(* Logix 5000 Rung export; software revision 16.04 *)

TYPE AFCESiteAlarms :   // Indicates if a meter has any alarms
STRUCT
   Meter1 : BOOL;   // Meter in alarm
   Meter2 : BOOL;   // Meter in alarm
   Meter3 : BOOL;   // Meter in alarm
   Meter4 : BOOL;   // Meter in alarm
   Meter5 : BOOL;   // Meter in alarm
   Meter6 : BOOL;   // Meter in alarm
   Meter7 : BOOL;   // Meter in alarm
   Meter8 : BOOL;   // Meter in alarm
   Meter9 : BOOL;   // Meter in alarm
   Meter10 : BOOL;   // Meter in alarm
   Meter11 : BOOL;   // Meter in alarm
   Meter12 : BOOL;   // Meter in alarm
   Meter13 : BOOL;   // Meter in alarm
   Meter14 : BOOL;   // Meter in alarm
   Meter15 : BOOL;   // Meter in alarm
   Meter16 : BOOL;   // Meter in alarm
END_STRUCT
END_TYPE

TYPE AFCEFlag :   // Flags contains status information updated by ladder and also trigger bits for clock update
STRUCT
   AFCStopped : BOOL;   // Indicates that the module has sent a new input block to be processed by ladder - UPDATED BY LADDER
   AFCInputSequenceNum : INT;   // Meter number (0 -15) associated to blocks 1-16. Used to update "Profile" (meter type and product group.) UPDATED BY LADDER
END_STRUCT
END_TYPE

TYPE AFCEUtilBlockNonInterrupt :
STRUCT
   Now : BOOL;
   ModbusMasterCommand : BOOL;
   ModbusMasterResponse : BOOL;
   Archive : DINT;
   Prover : BOOL;
   PassThru : BOOL;
   Calibration : BOOL;
END_STRUCT
END_TYPE

TYPE AFCEProveConfigEnable :   // Prove controls at enable
STRUCT
   MeterNumber : INT;   // Meter number requested (1-16)
   AutoAcceptProve : BOOL;   // Auto-accept the prove
   AutoContinueProve : BOOL;   // Auto-continue the prove
END_STRUCT
END_TYPE

TYPE AFCEModbusGateway :   // Modbus Gateway
STRUCT
   Command : AFCEModbusGatewayCommand[10];   // Modbus gateway commands - contains setup and modbus data
END_STRUCT
END_TYPE

TYPE AFCENetworkConfig :
STRUCT
   GatewayIndex : DINT;
   Physical_Interface_IP : INT[4];
   Physical_Interface_Network_Prefix : SINT;
   Default_Gateway_IP : INT[4];   // The IP address of the gateway. Must be in the same network as the web interface, or null.
   Server1_Network_Prefix : SINT;   // The network prefix length (number of subnet mask bits) of the interface for server 1; a number between 0 and 32.
   Server1_MBAP_Port : DINT;   // The Modbus-TCP port for server 1; 502, or a number between 1024 and 65535.
   Server1_Listener_IP : INT[4];   // The IP address of the network interface for server 1.
END_STRUCT
END_TYPE

TYPE AFCEModbusMasterDataType :   // Modbus master data type
STRUCT
   Bit : BOOL;   // bit type
   Word : BOOL;   // word type (16-bit)
   Long : BOOL;   // long integer (32-bit)
   LongRemote : BOOL;   // long integer (32-bit)
END_STRUCT
END_TYPE

TYPE AFCEUtil :   // Used for internal ladder logic usage. These values must not be changed by user application.
STRUCT
   Flags : AFCEFlag;   // Wallclock update commands
   CycleCounter : INT;   // Reflects current block ID calculated by ladder to be sent to the module
   Buffer : AFCEUtilBuffer;
   Block : AFCEUtilBlock;
END_STRUCT
END_TYPE

TYPE AFCEWallclock :
STRUCT
   GetAFCTime : BOOL;   // Get current AFC Time
   SetAFCTimeFromPLCTime : BOOL;   // Set AFC time from PLC time. Updates current AFC time
   EnableLocalDateTime : BOOL;   // Enable Local Date Time.
   AFCTime : AFCETime;   // Coordinated Universal Time. Updated by either getting or setting AFC time.
END_STRUCT
END_TYPE

TYPE AFCEProvePhaseBitmap :   // AFC prove phase bitmap
STRUCT
   NotSelected : BOOL;   // Not selected
   Active : BOOL;   // Active, not counting
   CountingPast1stSwitch : BOOL;   // Counting past 1st switch for Udir and forward leg for Bdir)
   Past2ndSwitchFwdLeg : BOOL;   // Past 2nd switch forward leg (bidirectional only)
   Past1stSwithRetLeg : BOOL;   // Past 1st switch return leg (bidirectional only)
   RunComplete : BOOL;   // Run complete. past 2nd switch.
END_STRUCT
END_TYPE

TYPE AFCEProveInputConfig :   // Prove input block results - prover configuration
STRUCT
   Type : INT;   // Prover type
   Options : INT;   // Prover options
   RunsPerProveTotal : INT;   // Total runs per prove
   RunsPerProveSelected : INT;   // Selected runs per prove
   MaxRunsBeforeAbort : INT;   // Max total runs before abort
   ShortPassesPerRun : INT;   // Short passes per run if bidir = 2 , else 0
END_STRUCT
END_TYPE

TYPE AFCEModbusGatewayCommand :   // Modbus Gateway Command
STRUCT
   Config : AFCEModbusGatewayConfig;   // Config data to be entered by the user.
   Trigger : BOOL;   // Trigger the Command, when cleared module has responded.
   Data : INT[200];   // Contains modbus data written to the module (write commands)
END_STRUCT
END_TYPE

TYPE AFCENetworkUTIL :
STRUCT
   State : INT;
   Buffer : SINT[240];
   TimeoutTimer : TIMER;
   TimeoutState : INT;
END_STRUCT
END_TYPE

TYPE AFCEProveConfigAccept :   // Prove controls at accept. If auto-accept is selected must be available at enable
STRUCT
   RequestedInterpolationPoint : INT;   // Requested interpolation point (0 nearest)
   ApplyMFChangeAllStreams : BOOL;   // Apply change in meter factor to all streams
   ApplyMFChangeCurve : BOOL;   // Apply change in meter factor to all curve points
   ApplyNewMF : BOOL;   // CApply new meter factor
END_STRUCT
END_TYPE

TYPE AFCEModbusMasterCommand :   // Modbus Master Command
STRUCT
   Config : AFCEModbusMasterConfig;   // Modbus Master Configuration
   ErrorCode : INT;   // Error Code associated to Modbus Master Command
   Pending : BOOL;   // Pending Modbus Master Command - waiting for Modbus Response
   ReturnedTransactionID : DINT;   // Changes to Config.TransactionID value when response has returned.
   Data : INT[100];   // Read or Write Data
END_STRUCT
END_TYPE

TYPE AFCEProveSequencing :   // AFC prove sequencing tag for phase selection and ball positioning
STRUCT
   Phase : AFCEProvePhaseBitmap;   // AFC phase sequencing
   BallPositionReady : BOOL;   // Ball position: Ready (Udir & Bdir only; fwd leg Bdir)
   BallPositionSealed : BOOL;   // Ball position: Sealed (Udir & Bdir only; fwd leg Bdir)
   BallPositionReadyBwdLeg : BOOL;   // Ball position: Ready bwd leg (Bdir only)
   BallPositionSealedBwdLeg : BOOL;   // Ball position: Sealed bwd leg (Bdir only)
END_STRUCT
END_TYPE

TYPE AFCEUtilBlockInterrupt :
STRUCT
   Now : BOOL;
   ModbusGateway : DINT;
   EnableDisable : BOOL;
   Analysis : DINT;
END_STRUCT
END_TYPE

TYPE AFCEUtilBlock :
STRUCT
   ProcessInput : INT;
   InterruptPending : AFCEUtilBlockInterrupt;
   InterruptComplete : AFCEUtilBlockInterrupt;
   NonInterruptPending : AFCEUtilBlockNonInterrupt;
   NonInterruptComplete : AFCEUtilBlockNonInterrupt;
END_STRUCT
END_TYPE

TYPE AFCEModbusGatewayConfig :   // Modbus Ggateway Configuration
STRUCT
   Enable : BOOL;   // Set to 1 to enable modbus gateway command (0=disable)
   StartRegister : DINT;   // Start modbus address
   RegisterCount : INT;   // Word count (200 max)
   FunctionType : BOOL;   // 0 = read command, 1 = write command
   RegisterType : BOOL;   // 0 = holding register, 1 = input register
   SlaveType : BOOL;   // 0 = primary slave, 1 = virtual slave
END_STRUCT
END_TYPE

TYPE AFCENetwork :
STRUCT
   Read : BOOL;   // Trigger to read network parameters
   Write : BOOL;   // Trigger to write network parameters
   Config : AFCENetworkConfig;   // Network parameters
   Error : INT;   // 0 = OK, -1 = Timeout, -2 = Gateway Index Out of Range
   Util : AFCENetworkUTIL;   // Internal variables
END_STRUCT
END_TYPE

TYPE AFCEModbusPassThru :   // AFC Modbus Pass-thru
STRUCT
   Enable : BOOL;   // Set to 1 to enable pass-thru functionality (requires AFC Manager setting)
   MessagePresent : BOOL;   // Message present in the response block
   GetMessage : BOOL;   // Get the pass-thru message. When the bit is cleared the message has been transferred to the PLC.
   FunctionBitWrite : BOOL;   // Function bit write
   OverflowError : BOOL;   // Overflow error flag
   ModbusAddress : INT;   // Destination modbus address
   RegisterCount : INT;   // Number of elements associated to command
   ReadDataWord : INT[125];   // Contains received data for word commands
   ReadDataBit : AFCEModbusPassThruBitData;   // Contains received data for bit commands
END_STRUCT
END_TYPE

TYPE AFCEUtilBuffer :   // Buffer
STRUCT
   Input : INT[248];   // Input buffer contains the complete block to be copied from the module
   Output : INT[247];   // Output buffer contains data the complete block to be copied to the module
   Process : INT[180];
   ArchiveDay : INT[98];
   ArchiveHour : INT[98];
   Prove : INT[26];
   Analysis : INT[198];
   MeterEnableDisable : INT[4];
   StreamEnable : INT[36];
   StreamDisable : INT[36];
   StreamSelect : INT[24];
   MeterSignals : INT[24];
   Calibration : INT[36];
END_STRUCT
END_TYPE

TYPE AFCEProveStatus :   // Status of the prove (returned from the module to the processor)
STRUCT
   ProveAccepted : BOOL;   // Prove was accepted
   MeterFactorApplied : BOOL;   // Meter factor was applied
   MFAppliedToCurve : BOOL;   // Meter factor was applied to all points in the curve
   MFAppliedToStreams : BOOL;   // Meter factor was applied to all streams
   ProveRejectedByCommand : BOOL;   // Prove was rejected by command
   ProveRejectedNoRuns : BOOL;   // Prove was rejected - empty prove (no runs)
   ProveRejectedDivideBy0 : BOOL;   // Prove was rejected - divide by 0
   ProveEnabled : BOOL;   // Prove is enabled
   ProvingRunInProgress : BOOL;   // Proving run is in progress
   ProveRejectedAbort : BOOL;   // Prove rejected: abort
   ProvePaused : BOOL;   // Prove is paused
   RunCancelled : BOOL;   // Run Is cancelled
   RunTimedOut : BOOL;   // Run timed out
END_STRUCT
END_TYPE

TYPE AFCEProveConfig :   // Controls (configuration settings) associated to the prover
STRUCT
   Enable : AFCEProveConfigEnable;   // Controls at enable
   Accept : AFCEProveConfigAccept;   // Controls at accept
END_STRUCT
END_TYPE

TYPE AFCESiteStatus :   // Site status bits - contains general information about the module - not meter specific
STRUCT
   AFCActive : BOOL;   // AFC active
   ChecksumAlarms : BOOL;   // Checkum alarm active
   Reserved2 : BOOL;
   Reserved3 : BOOL;
   PLCHalted : BOOL;   // PLC in program mode or missing
   CfgChanged : BOOL;   // Configuration changed
   Powerup : BOOL;   // Module powered up
   ColdStart : BOOL;   // Module performed cold start (BBRAM initialized)
   ModbusMasterPending : BOOL;   // Modbus Master Poll Pending
   ModbusMasterComplete : BOOL;   // Modbus Master Poll Complete
   ModbusPassThruPending : BOOL;   // Modbus Pass-thru Input Pending
   CalibrationRequest : BOOL;   // Calibration request from module
   ProverEnabled : BOOL;   // Prover Enabled
   Reserved13 : BOOL;
   Reserved14 : BOOL;
   Reserved15 : BOOL;
END_STRUCT
END_TYPE

TYPE AFCEModbusMaster :   // Modbus Master. Port 3 must be configured as modbus master through AFC Manager to use this feature.
STRUCT
   Enable : BOOL;   // Enable the modbus master funcionality
   CommandIndex : INT;   // Selects which command index will be executed
   Command : AFCEModbusMasterCommand[10];   // Each command contains a specific modbus request to be sent out of the port
END_STRUCT
END_TYPE

TYPE AFCEProveProcess :   // Prove process output from processor to the module
STRUCT
   Sequencing : AFCEProveSequencing;   // Prover sequencing
   Temperature : REAL;   // Temperature for Single Probe provers. And Inlet Temperature for Dual Probe Provers.
   OutletTemperature : REAL;   // Outlet Temperature for Provers with Dual Probes.
   SwitchBarTemperature : REAL;   // Switch bar temperature
   Pressure : REAL;   // Pressure for Single Probe provers. And Inlet Pressure for Dual Probe Provers.
   OutletPressure : REAL;   // Outlet Pressure for Provers with Dual Probes.
   ProverDensity : REAL;   // Prover density
END_STRUCT
END_TYPE

TYPE AFCETime :   // AFC time format used for wallclock update.
STRUCT
   Year : DINT;   // Year
   Month : DINT;   // Month
   Day : DINT;   // Day
   Hour : DINT;   // Hour
   Minute : DINT;   // Minute
   second : DINT;   // Seconds
END_STRUCT
END_TYPE

TYPE AFCEModbusMasterSwap :   // Modbus master swap words/ swap bytes
STRUCT
   SwapWords : BOOL;   // Swap words
   SwapBytes : BOOL;   // Swap bytes
END_STRUCT
END_TYPE

TYPE AFCEProvePulseCount :   // Values to be supplied at the end of the pass/run
STRUCT
   Meter : DINT;   // Meter pulse count
   MasterMeter : DINT;   // Master meter pulse count
END_STRUCT
END_TYPE

TYPE AFCEModbusPassThruBitData :   // AFC Modbus Pass-thru Bit Data
STRUCT
   Data : BOOL[2016];   // Contains received data for bit commands
END_STRUCT
END_TYPE

TYPE AFCEModbusMasterConfig :   // Modbus master command settings
STRUCT
   Enable : BOOL;   // Set to 1 to enable command (0=disable)
   FunctionType : BOOL;   // Set to 1 to select write command (0=read command)
   RegisterBank : BOOL;   // Set to 1 to select input register (0=holding register)
   DataType : AFCEModbusMasterDataType;   // Select data type format
   SwapOption : AFCEModbusMasterSwap;   // Select byte and word swap (1 = swap, 0 = no swap)
   TypeSwap : INT;   // This value is calculated by ladder logic and must not be modified by user
   SlaveAddress : INT;   // Modbus slave address of remote device
   ModbusAddress : INT;   // Modbus data address on remote slave
   ElementCount : INT;   // Number of data elements (125 words)
   TransactionID : INT;   // Transaction ID. This value is returned to the ReturnedTransaction ID when the response has been received.
END_STRUCT
END_TYPE

TYPE AFCEModuleDef :   // Main user defined data type
STRUCT
   ModbusGateway : AFCEModbusGateway;   // Reads and write data between processor and module modbus table
   ModbusMaster : AFCEModbusMaster;   // Setup modbus master commands to be sent to remote slaves (through Port 3)
   ModbusPassThru : AFCEModbusPassThru;   // Modbus pass-thru data
   SiteStatus : AFCESiteStatus;   // Site status
   MeterAlarms : AFCESiteAlarms;   // Meter Alarms
   Prove : AFCEProve;   // Prover
   Wallclock : AFCEWallclock;   // Set clock and get clock information
   Firmware : AFCEFirmwareVersion;   // Firmware information
   Util : AFCEUtil;   // Used by ladder logic
END_STRUCT
END_TYPE

TYPE AFCEProveSignals :   // Contains the proving signals that will trigger specific tasks from the module
STRUCT
   EnableProve : BOOL;   // Enables the prove
   AcceptProve : BOOL;   // Accepts the prove
   RejectProve : BOOL;   // Reject the prove
   RunStart : BOOL;   // Starts the run
   RunComplete : BOOL;   // Flags that the run is complete
   RunCancel : BOOL;   // Cancels the run
   RunDelete : BOOL;   // Deletes the run
   PassComplete : BOOL;   // Flag that the pass is complete
   PauseProve : BOOL;   // Pauses the Proving Process
   AbortProve : BOOL;   // Aborts the prove
END_STRUCT
END_TYPE

TYPE AFCEFirmwareVersion :
STRUCT
   Major : SINT;   // Major Version number
   Minor : SINT;   // Minor Version number
   Revision : INT;   // Revision
END_STRUCT
END_TYPE

TYPE AFCEProveRunResults :   // Run results of the prove. Copied from the module to the pocessor
STRUCT
   CountAttempted : INT;   // Run count attempted
   CountCompleted : INT;   // Run count completed
   CountSelected : INT;   // Run count selected
   RunsSelected : INT;   // Bit Mapped Runs selected for calculations from completed runs
   NewMeterFactor : REAL;   // New meter factor
   ChangeInMeterFactor : REAL;   // Change in meter factor
END_STRUCT
END_TYPE

TYPE AFCEProve :   // Prove
STRUCT
   Process : AFCEProveProcess;   // Process Variables
   Signals : AFCEProveSignals;   // AFC Prove Signals (triggers the proving update)
   Config : AFCEProveConfig;   // AFC Prove Control (configuration settings)
   PulseCounts : AFCEProvePulseCount;   // Pulse counts to be updated at the end of the run/pass
   ConfigInput : AFCEProveInputConfig;   // AFC prover input configuration
   Status : AFCEProveStatus;   // AFC prover status
   ErrorCode : INT;   // Prove error code
   ProveControlsEcho : INT;   // AFC module Echos the state of the Prove Controls
   RequestedMeterEcho : INT;   // AFC module Echos the Meter number requested
   RequestedCurvePointEcho : INT;   // AFC module Echos the requested Curve Point
   RunResults : AFCEProveRunResults;   // Prove and run results
   ProveEnabled : BOOL;   // ON if prove is enabled. This flag is coped from inputbuffer[247]
END_STRUCT
END_TYPE

ADD_ON_INSTRUCTION AOI69EAFCNetworkConfig   (* revision 1.0, ExecutePrescan *)
// Add-On instruction to update the MVI69E-AFC network settings
// Revision note:
// Read and write module network configuration.
// Help:
// v1.0 Read and write module network configuration.
VAR_IN_OUT
   Network : AFCENetwork; {required}
   EAFC : AFCEModuleDef; {required}
END_VAR
VAR
   NetworkBuffer : DINT[2];
   MVMbuffer : INT;
   IndexSizeM1 : DINT;
   IndexSize : DINT;
   Index : DINT;
   ErrorTimer : TIMER;
END_VAR

ROUTINE Logic   (* ladder *)
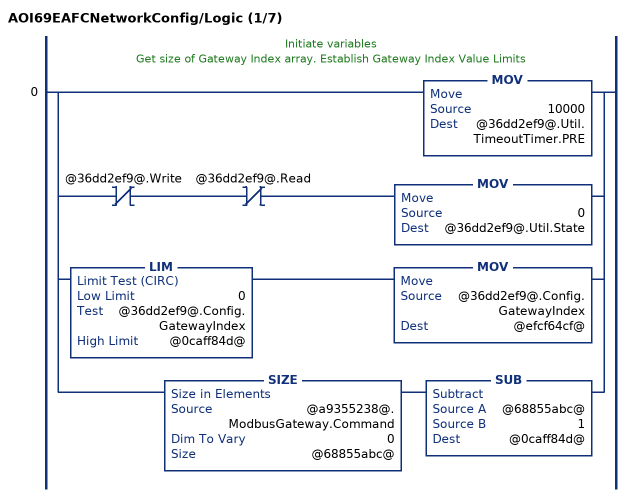
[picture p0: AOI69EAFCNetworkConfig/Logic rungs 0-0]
   // Initiate variables
   // Get size of Gateway Index array. Establish Gateway Index Value Limits
   0: [[MOV(10000,@36dd2ef9@.Util.TimeoutTimer.PRE) ,XIO(@36dd2ef9@.Write) XIO(@36dd2ef9@.Read) MOV(0,@36dd2ef9@.Util.State) ] ,LIM(0,@36dd2ef9@.Config.GatewayIndex,@0caff84d@) MOV(@36dd2ef9@.Config.GatewayIndex,@efcf64cf@) ,SIZE(@a9355238@.ModbusGateway.Command,0,@68855abc@) SUB(@68855abc@,1,@0caff84d@) ];
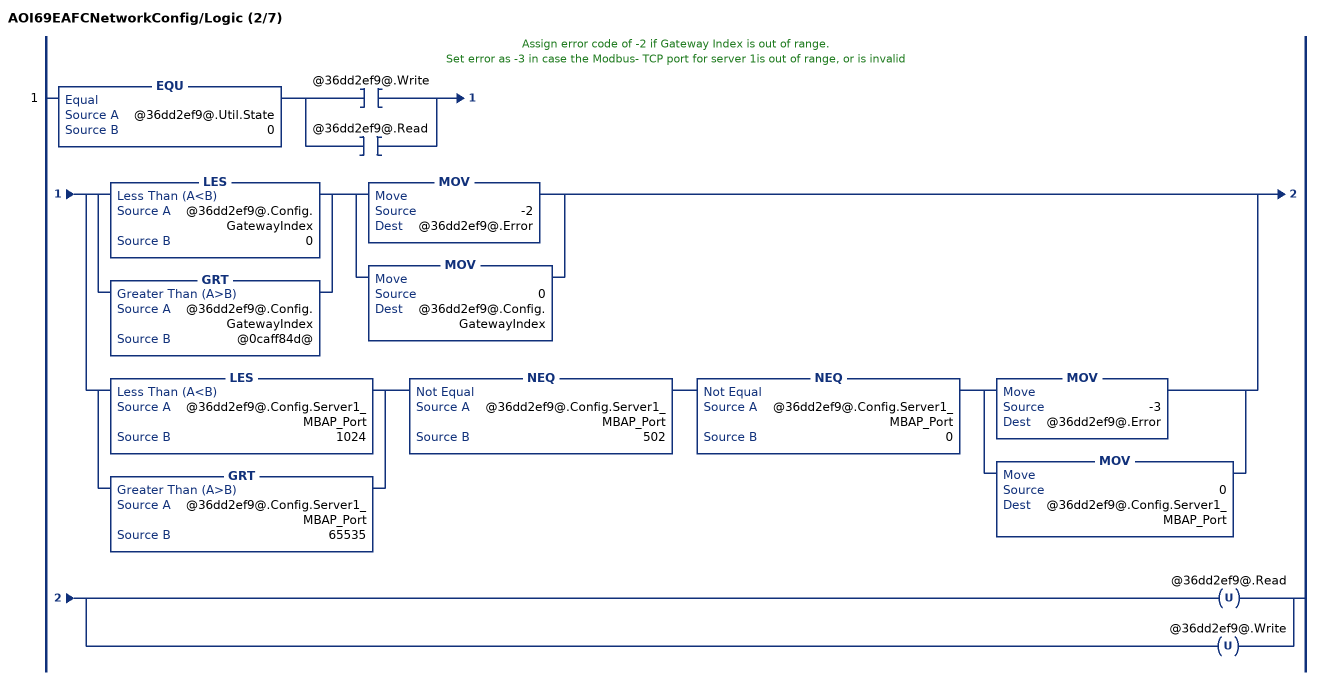
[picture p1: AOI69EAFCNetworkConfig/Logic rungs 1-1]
   // Assign error code of -2 if Gateway Index is out of range.
   // Set error as -3 in case the Modbus- TCP port for server 1is out of range, or is invalid
   1: EQU(@36dd2ef9@.Util.State,0)[XIC(@36dd2ef9@.Write) ,XIC(@36dd2ef9@.Read) ][[LES(@36dd2ef9@.Config.GatewayIndex,0) ,GRT(@36dd2ef9@.Config.GatewayIndex,@0caff84d@) ] [MOV(-2,@36dd2ef9@.Error) ,MOV(0,@36dd2ef9@.Config.GatewayIndex) ] ,[LES(@36dd2ef9@.Config.Server1_MBAP_Port,1024) ,GRT(@36dd2ef9@.Config.Server1_MBAP_Port,65535) ] NEQ(@36dd2ef9@.Config.Server1_MBAP_Port,502) NEQ(@36dd2ef9@.Config.Server1_MBAP_Port,0) [MOV(-3,@36dd2ef9@.Error) ,MOV(0,@36dd2ef9@.Config.Server1_MBAP_Port) ] ][OTU(@36dd2ef9@.Read) ,OTU(@36dd2ef9@.Write) ];
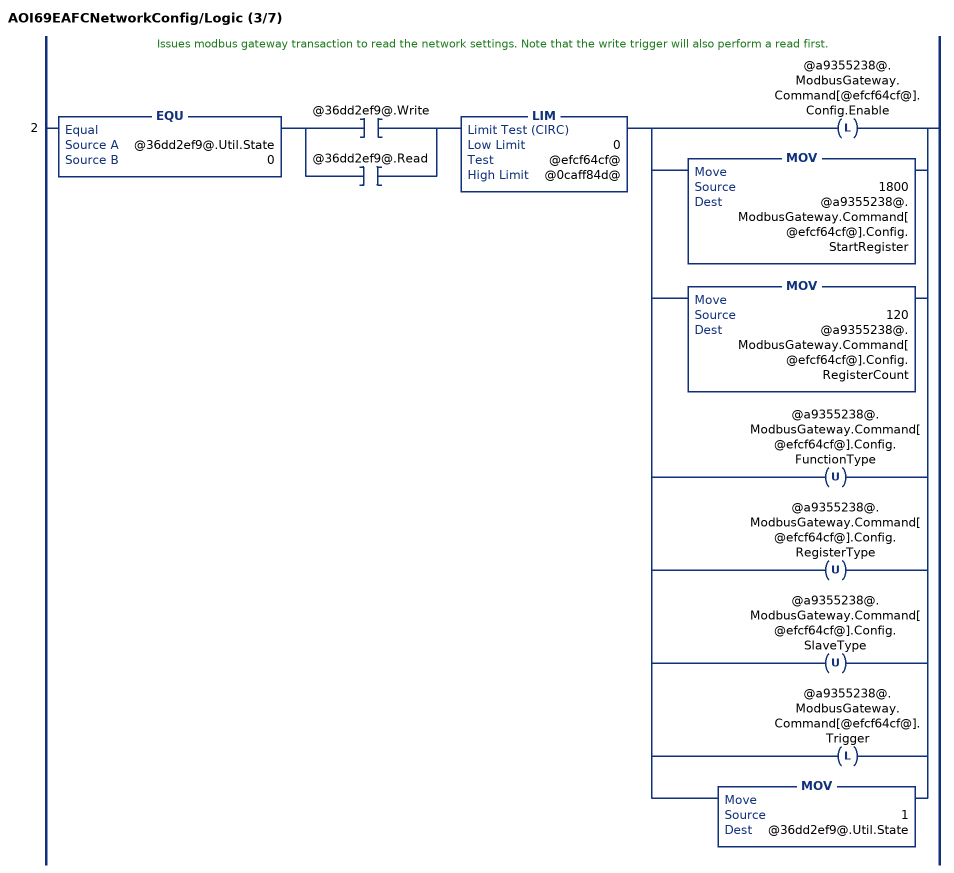
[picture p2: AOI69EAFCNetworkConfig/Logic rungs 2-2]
   // Issues modbus gateway transaction to read the network settings. Note that the write trigger will also perform a read first.
   2: EQU(@36dd2ef9@.Util.State,0)[XIC(@36dd2ef9@.Write) ,XIC(@36dd2ef9@.Read) ]LIM(0,@efcf64cf@,@0caff84d@)[OTL(@a9355238@.ModbusGateway.Command[@efcf64cf@].Config.Enable) ,MOV(1800,@a9355238@.ModbusGateway.Command[@efcf64cf@].Config.StartRegister) ,MOV(120,@a9355238@.ModbusGateway.Command[@efcf64cf@].Config.RegisterCount) ,OTU(@a9355238@.ModbusGateway.Command[@efcf64cf@].Config.FunctionType) ,OTU(@a9355238@.ModbusGateway.Command[@efcf64cf@].Config.RegisterType) ,OTU(@a9355238@.ModbusGateway.Command[@efcf64cf@].Config.SlaveType) ,OTL(@a9355238@.ModbusGateway.Command[@efcf64cf@].Trigger) ,MOV(1,@36dd2ef9@.Util.State) ];
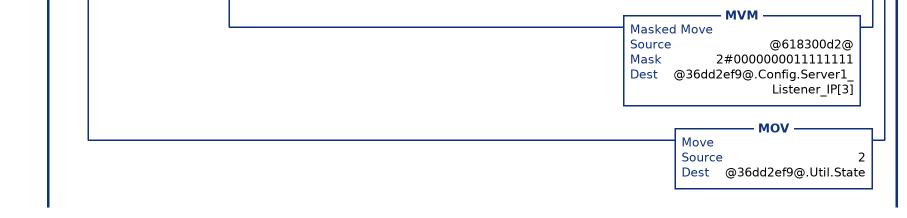
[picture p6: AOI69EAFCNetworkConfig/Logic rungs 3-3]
   // Parses the data received from the module once it detects that the gateway transaction was concluded.
   3: EQU(@36dd2ef9@.Util.State,1)[XIC(@36dd2ef9@.Write) ,XIC(@36dd2ef9@.Read) ]XIO(@a9355238@.ModbusGateway.Command[@efcf64cf@].Trigger)LIM(0,@efcf64cf@,@0caff84d@)[COP(@a9355238@.ModbusGateway.Command[@efcf64cf@].Data[0],@36dd2ef9@.Util.Buffer[0],240) ,XIC(@36dd2ef9@.Read) [COP(@36dd2ef9@.Util.Buffer[3],@618300d2@,1) ,MVM(@618300d2@,2#0000000011111111,@36dd2ef9@.Config.Physical_Interface_IP[0]) ,COP(@36dd2ef9@.Util.Buffer[2],@618300d2@,1) ,MVM(@618300d2@,2#0000000011111111,@36dd2ef9@.Config.Physical_Interface_IP[1]) ,COP(@36dd2ef9@.Util.Buffer[1],@618300d2@,1) ,MVM(@618300d2@,2#0000000011111111,@36dd2ef9@.Config.Physical_Interface_IP[2]) ,COP(@36dd2ef9@.Util.Buffer[0],@618300d2@,1) ,MVM(@618300d2@,2#0000000011111111,@36dd2ef9@.Config.Physical_Interface_IP[3]) ,MOV(@36dd2ef9@.Util.Buffer[4],@36dd2ef9@.Config.Physical_Interface_Network_Prefix) ,COP(@36dd2ef9@.Util.Buffer[15],@618300d2@,1) ,MVM(@618300d2@,2#0000000011111111,@36dd2ef9@.Config.Default_Gateway_IP[0]) ,COP(@36dd2ef9@.Util.Buffer[14],@618300d2@,1) ,MVM(@618300d2@,2#0000000011111111,@36dd2ef9@.Config.Default_Gateway_IP[1]) ,COP(@36dd2ef9@.Util.Buffer[13],@618300d2@,1) ,MVM(@618300d2@,2#0000000011111111,@36dd2ef9@.Config.Default_Gateway_IP[2]) ,COP(@36dd2ef9@.Util.Buffer[12],@618300d2@,1) ,MVM(@618300d2@,2#0000000011111111,@36dd2ef9@.Config.Default_Gateway_IP[3]) ,MOV(@36dd2ef9@.Util.Buffer[20],@36dd2ef9@.Config.Server1_Network_Prefix) ,COP(@36dd2ef9@.Util.Buffer[26],@38ffdbdb@[0],2) MVM(@38ffdbdb@[0],2#00000000000000001111111111111111,@36dd2ef9@.Config.Server1_MBAP_Port) ,COP(@36dd2ef9@.Util.Buffer[31],@618300d2@,1) ,MVM(@618300d2@,2#0000000011111111,@36dd2ef9@.Config.Server1_Listener_IP[0]) ,COP(@36dd2ef9@.Util.Buffer[30],@618300d2@,1) ,MVM(@618300d2@,2#0000000011111111,@36dd2ef9@.Config.Server1_Listener_IP[1]) ,COP(@36dd2ef9@.Util.Buffer[29],@618300d2@,1) ,MVM(@618300d2@,2#0000000011111111,@36dd2ef9@.Config.Server1_Listener_IP[2]) ,COP(@36dd2ef9@.Util.Buffer[28],@618300d2@,1) ,MOV(0,@36dd2ef9@.Error) ,MVM(@618300d2@,2#0000000011111111,@36dd2ef9@.Config.Server1_Listener_IP[3]) ] ,MOV(2,@36dd2ef9@.Util.State) ];
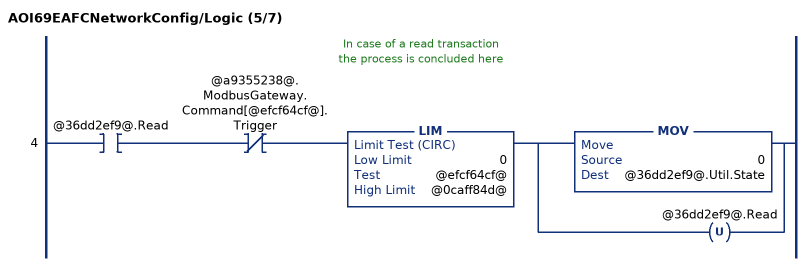
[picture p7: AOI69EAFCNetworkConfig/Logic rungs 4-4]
   // In case of a read transaction
   //  the process is concluded here
   4: XIC(@36dd2ef9@.Read)XIO(@a9355238@.ModbusGateway.Command[@efcf64cf@].Trigger)LIM(0,@efcf64cf@,@0caff84d@)[MOV(0,@36dd2ef9@.Util.State) ,OTU(@36dd2ef9@.Read) ];
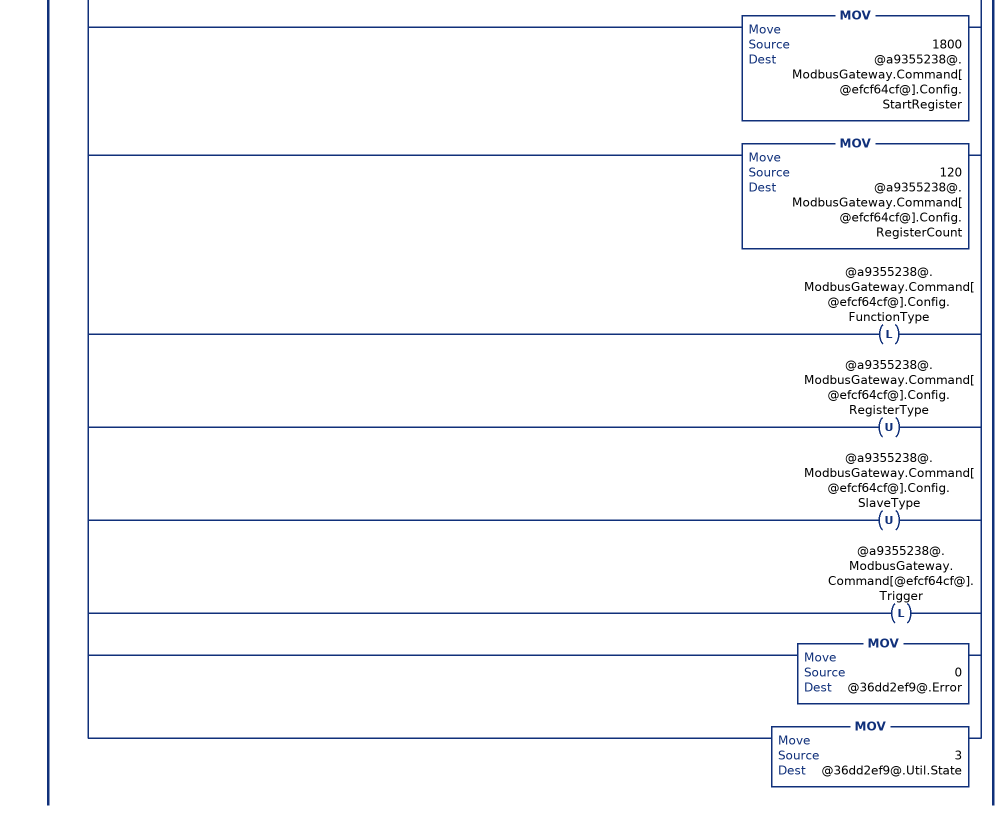
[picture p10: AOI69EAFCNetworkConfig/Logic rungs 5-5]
   // In case this is a write transaction
   //  this rung will update the the specific parameters listed at Network.Config and keep the remaining data the same as read from the module.
   5: EQU(@36dd2ef9@.Util.State,2)[LIM(1024,@36dd2ef9@.Config.Server1_MBAP_Port,65535) ,EQU(@36dd2ef9@.Config.Server1_MBAP_Port,502) ]LIM(0,@efcf64cf@,@0caff84d@)XIC(@36dd2ef9@.Write)[COP(@36dd2ef9@.Config.Physical_Interface_IP[0],@36dd2ef9@.Util.Buffer[3],1) ,COP(@36dd2ef9@.Config.Physical_Interface_IP[1],@36dd2ef9@.Util.Buffer[2],1) ,COP(@36dd2ef9@.Config.Physical_Interface_IP[2],@36dd2ef9@.Util.Buffer[1],1) ,COP(@36dd2ef9@.Config.Physical_Interface_IP[3],@36dd2ef9@.Util.Buffer[0],1) ,MOV(@36dd2ef9@.Config.Physical_Interface_Network_Prefix,@36dd2ef9@.Util.Buffer[4]) ,COP(@36dd2ef9@.Config.Default_Gateway_IP[0],@36dd2ef9@.Util.Buffer[15],1) ,COP(@36dd2ef9@.Config.Default_Gateway_IP[1],@36dd2ef9@.Util.Buffer[14],1) ,COP(@36dd2ef9@.Config.Default_Gateway_IP[2],@36dd2ef9@.Util.Buffer[13],1) ,COP(@36dd2ef9@.Config.Default_Gateway_IP[3],@36dd2ef9@.Util.Buffer[12],1) ,MOV(@36dd2ef9@.Config.Server1_Network_Prefix,@36dd2ef9@.Util.Buffer[20]) ,COP(@36dd2ef9@.Config.Server1_MBAP_Port,@36dd2ef9@.Util.Buffer[26],2) ,COP(@36dd2ef9@.Config.Server1_Listener_IP[0],@36dd2ef9@.Util.Buffer[31],1) ,COP(@36dd2ef9@.Config.Server1_Listener_IP[1],@36dd2ef9@.Util.Buffer[30],1) ,COP(@36dd2ef9@.Config.Server1_Listener_IP[2],@36dd2ef9@.Util.Buffer[29],1) ,COP(@36dd2ef9@.Config.Server1_Listener_IP[3],@36dd2ef9@.Util.Buffer[28],1) ,COP(@36dd2ef9@.Util.Buffer[0],@a9355238@.ModbusGateway.Command[@efcf64cf@].Data[0],120) ,MOV(1800,@a9355238@.ModbusGateway.Command[@efcf64cf@].Config.StartRegister) ,MOV(120,@a9355238@.ModbusGateway.Command[@efcf64cf@].Config.RegisterCount) ,OTL(@a9355238@.ModbusGateway.Command[@efcf64cf@].Config.FunctionType) ,OTU(@a9355238@.ModbusGateway.Command[@efcf64cf@].Config.RegisterType) ,OTU(@a9355238@.ModbusGateway.Command[@efcf64cf@].Config.SlaveType) ,OTL(@a9355238@.ModbusGateway.Command[@efcf64cf@].Trigger) ,MOV(0,@36dd2ef9@.Error) ,MOV(3,@36dd2ef9@.Util.State) ];
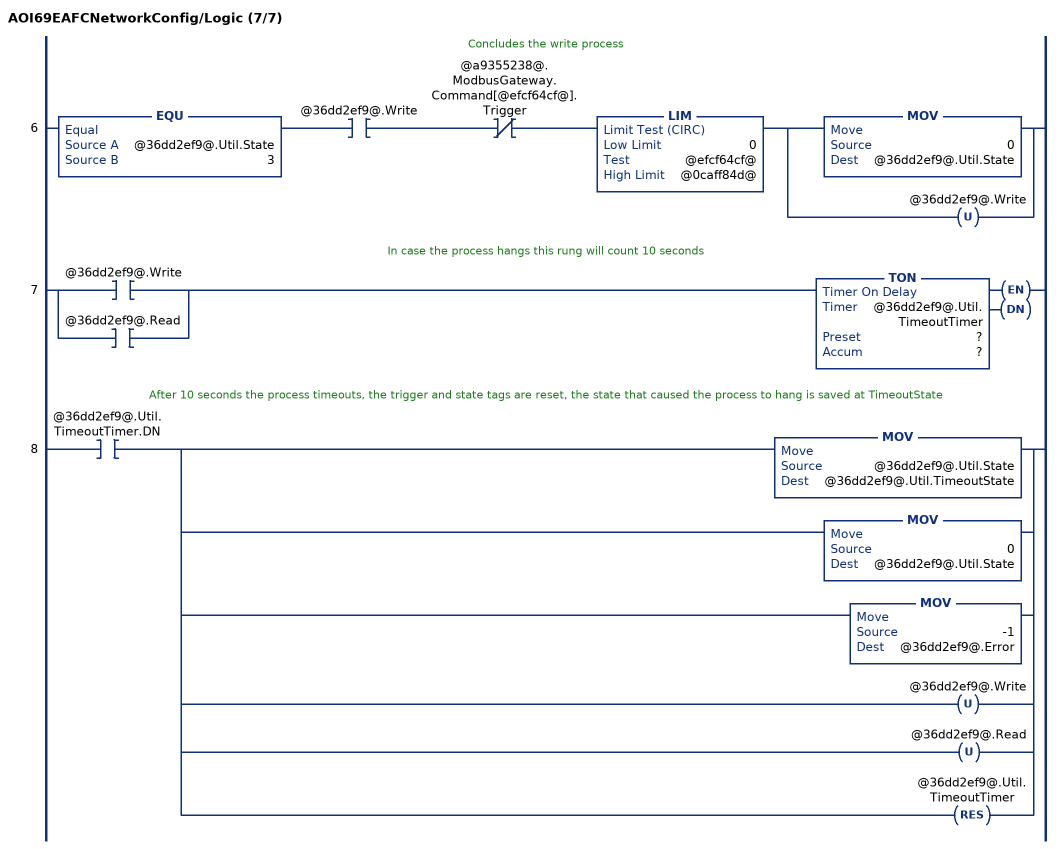
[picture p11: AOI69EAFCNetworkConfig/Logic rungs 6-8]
   // Concludes the write process
   6: EQU(@36dd2ef9@.Util.State,3)XIC(@36dd2ef9@.Write)XIO(@a9355238@.ModbusGateway.Command[@efcf64cf@].Trigger)LIM(0,@efcf64cf@,@0caff84d@)[MOV(0,@36dd2ef9@.Util.State) ,OTU(@36dd2ef9@.Write) ];
   // In case the process hangs this rung will count 10 seconds
   7: [XIC(@36dd2ef9@.Write) ,XIC(@36dd2ef9@.Read) ]TON(@36dd2ef9@.Util.TimeoutTimer,?,?);
   // After 10 seconds the process timeouts, the trigger and state tags are reset, the state that caused the process to hang is saved at TimeoutState
   8: XIC(@36dd2ef9@.Util.TimeoutTimer.DN)[MOV(@36dd2ef9@.Util.State,@36dd2ef9@.Util.TimeoutState) ,MOV(0,@36dd2ef9@.Util.State) ,MOV(-1,@36dd2ef9@.Error) ,OTU(@36dd2ef9@.Write) ,OTU(@36dd2ef9@.Read) ,RES(@36dd2ef9@.Util.TimeoutTimer) ];
END_ROUTINE

ROUTINE Prescan   (* ladder *)
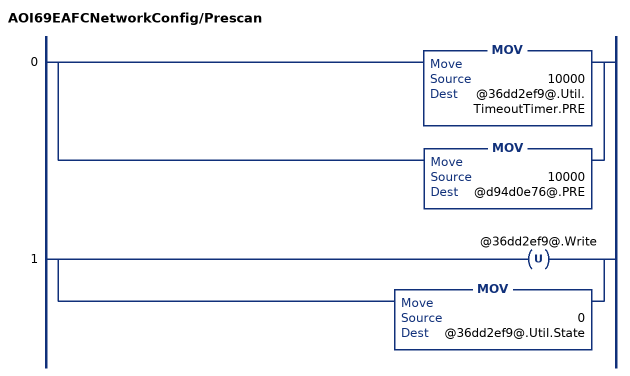
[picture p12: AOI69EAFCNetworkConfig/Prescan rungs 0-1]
   0: [MOV(10000,@36dd2ef9@.Util.TimeoutTimer.PRE) ,MOV(10000,@d94d0e76@.PRE) ];
   1: [OTU(@36dd2ef9@.Write) ,MOV(0,@36dd2ef9@.Util.State) ];
END_ROUTINE
END_ADD_ON_INSTRUCTION

VAR_GLOBAL   (* controller tags *)
   AFC : AFCEModuleDef;
   AOINetworkConfig : AOI69EAFCNetworkConfig;
   Network : AFCENetwork;
END_VAR

PROGRAM MainProgram

ROUTINE MainRoutine   (* ladder *)
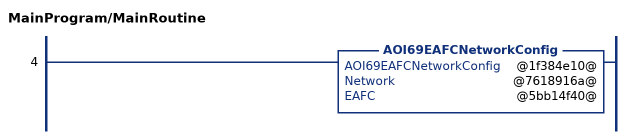
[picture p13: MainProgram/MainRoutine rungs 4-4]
   4: AOI69EAFCNetworkConfig(@1f384e10@,@7618916a@,@5bb14f40@);
END_ROUTINE
END_PROGRAM
